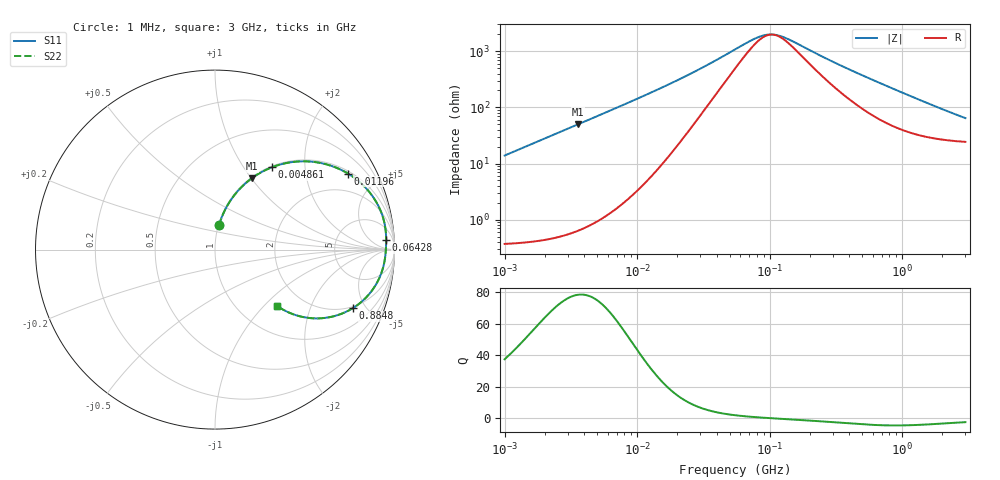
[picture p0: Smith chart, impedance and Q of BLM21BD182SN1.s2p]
! BLM21BD182SN1
# Hz S RI R 50
!Freq.(Hz) S11(Real) S11(Imag) S21(Real) S21(Imag) S12(Real) S12(Imag) S22(Real) S22(Imag)
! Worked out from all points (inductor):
!   401 points, 1 MHz to 3 GHz, reference 50 ohm
!   read as one part in series: L = 2.21 uH near 1.041 MHz
!   highest Q = 78.4 at 3.6 MHz (marker M1), where L = 2.22 uH
!   self-resonance near 105.1 MHz
!   S11 on the Smith chart (normalised r, x): 1 MHz: 1.01, +0.28; 4.861 MHz: 1.02, +1.36; 11.96 MHz: 1.10, +3.44; 64.28 MHz: 17, +21; 884.8 MHz: 1.89, -4.06; 3 GHz: 1.49, -1.19
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1000000  0.0224 0.1354  0.9776 -0.1354  0.9776 -0.1354  0.0224 0.1354
2055611  0.079 0.2622  0.921 -0.2622  0.921 -0.2622  0.079 0.2622
3600306  0.2043 0.3968  0.7957 -0.3968  0.7957 -0.3968  0.2043 0.3968
3823119  0.2243 0.4108  0.7757 -0.4108  0.7757 -0.4108  0.2243 0.4108
4861065  0.3181 0.4592  0.6819 -0.4592  0.6819 -0.4592  0.3181 0.4592
7550455  0.5304 0.4906  0.4696 -0.4906  0.4696 -0.4906  0.5304 0.4906
1.196486e7  0.7411 0.4237  0.2589 -0.4237  0.2589 -0.4237  0.7411 0.4237
1.461624e7  0.8102 0.3729  0.1898 -0.3729  0.1898 -0.3729  0.8102 0.3729
1.896016e7  0.8755 0.3007  0.1245 -0.3007  0.1245 -0.3007  0.8755 0.3007
2.559965e7  0.9208 0.2211  0.0792 -0.2211  0.0792 -0.2211  0.9208 0.2211
5.477226e7  0.9532 0.0757  0.0468 -0.0757  0.0468 -0.0757  0.9532 0.0757
6.428402e7  0.9537 0.0546  0.0463 -0.0546  0.0463 -0.0546  0.9537 0.0546
8.679508e7  0.953 0.0201  0.047 -0.0201  0.047 -0.0201  0.953 0.0201
1.081723e8  0.9518 -0.00302  0.0482 0.00302  0.0482 0.00302  0.9518 -0.00302
1.348146e8  0.9499 -0.0259  0.0501 0.0259  0.0501 0.0259  0.9499 -0.0259
2.094008e8  0.9424 -0.0759  0.0576 0.0759  0.0576 0.0759  0.9424 -0.0759
4.480278e8  0.8973 -0.1938  0.1027 0.1938  0.1027 0.1938  0.8973 -0.1938
8.005644e8  0.7942 -0.3085  0.2058 0.3085  0.2058 0.3085  0.7942 -0.3085
8.848309e8  0.7669 -0.3269  0.2331 0.3269  0.2331 0.3269  0.7669 -0.3269
1.218836e9  0.6614 -0.3714  0.3386 0.3714  0.3386 0.3714  0.6614 -0.3714
1.613037e9  0.5547 -0.3832  0.4453 0.3832  0.4453 0.3832  0.5547 -0.3832
3e9  0.3463 -0.3137  0.6537 0.3137  0.6537 0.3137  0.3463 -0.3137
